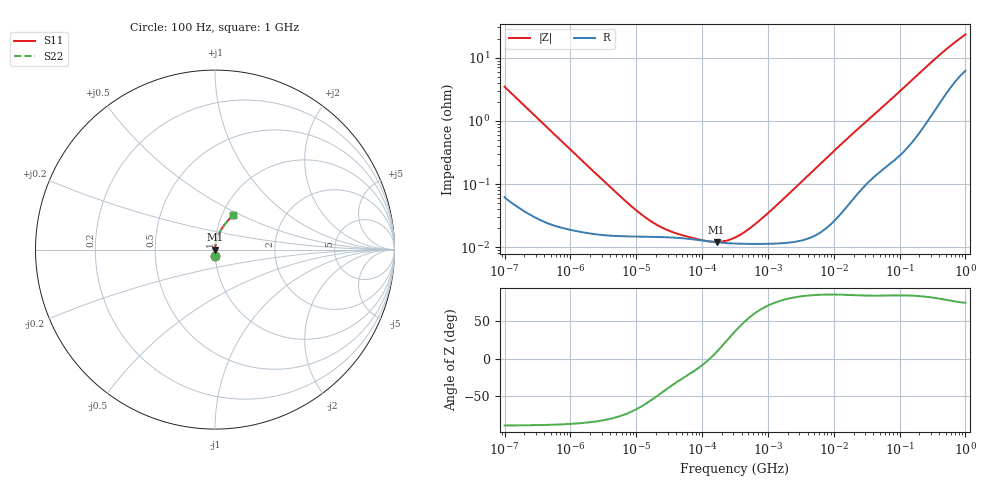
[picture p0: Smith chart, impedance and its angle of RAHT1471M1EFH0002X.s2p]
! RAHT1471M1EFH0002X  S-PARAMETER MODEL  (AEC-Q200 qualified)
! Model Generated by ELNA Corporation (http://www.ty-top.com)
! Version 1.0
! ELNA Control No. 201214
! Copyright (c) 2020 ELNA CO.,LTD. All Rights Reserved.
! Products Name : CONDUCTIVE POLYMER HYBRID ALUMINUM ELECTROLYTIC CAPACITORS
! Characteristics :
!  Capacitance  :  470uF  ,  Rated voltage  :  16V
!  Operating Temp. Range  :  -55 to +105 degC  ,  Endurance  :  5000hr at 105 degC
!  Dimension D  :  10mm  ,  Dimension L  :  10mm
! Frequency Range : 100Hz - 1GHz
! External Node Assignments :
!  1  o---| |---o  2
# MHz S RI R 50
!Freq[MHz].  S11 Real  S11 Imag  S21 Real  S21 Imag  S12 Real  S12 Imag  S22 Real  S22 Imag
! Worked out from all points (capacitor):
!   401 points, 100 Hz to 1 GHz, reference 50 ohm
!   read as one part in series: C = 461 uF near 108 Hz
!   lowest |Z| = 12.2 mohm at 166 kHz (marker M1)
!   series resonance near 131.1 kHz, so ESL is about 3.2 nH
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0.0001  0.00181 -0.0344  0.9982 0.0344  0.9982 0.0344  0.00181 -0.0344
0.000113  0.00149 -0.0305  0.9985 0.0305  0.9985 0.0305  0.00149 -0.0305
0.001488  0.000179 -0.00237  0.9998 0.00237  0.9998 0.00237  0.000179 -0.00237
0.00876  0.000148 -0.000406  0.9999 0.000406  0.9999 0.000406  0.000148 -0.000406
0.014207  0.000147 -0.00025  0.9999 0.00025  0.9999 0.00025  0.000147 -0.00025
0.022131  0.000146 -0.000161  0.9999 0.000161  0.9999 0.000161  0.000146 -0.000161
0.033113  0.000143 -0.000107  0.9999 0.000107  0.9999 0.000107  0.000143 -0.000107
0.055911  0.000138 -6.05e-05  0.9999 6.05e-05  0.9999 6.05e-05  0.000138 -6.05e-05
0.110917  0.000126 -1.24e-05  0.9999 1.24e-05  0.9999 1.24e-05  0.000126 -1.24e-05
0.165959  0.00012 1.9e-05  0.9999 -1.9e-05  0.9999 -1.9e-05  0.00012 1.9e-05
0.229087  0.000117 4.87e-05  0.9999 -4.87e-05  0.9999 -4.87e-05  0.000117 4.87e-05
0.316228  0.000115 8.49e-05  0.9999 -8.49e-05  0.9999 -8.49e-05  0.000115 8.49e-05
0.473151  0.000113 0.000144  0.9999 -0.000144  0.9999 -0.000144  0.000113 0.000144
0.767361  0.000113 0.000248  0.9999 -0.000248  0.9999 -0.000248  0.000113 0.000248
1.462177  0.000116 0.000484  0.9999 -0.000484  0.9999 -0.000484  0.000116 0.000484
4.704354  0.000148 0.00157  0.9999 -0.00157  0.9999 -0.00157  0.000148 0.00157
17.08048  0.000514 0.00553  0.9995 -0.00553  0.9995 -0.00553  0.000514 0.00553
69.9842  0.00246 0.0205  0.9975 -0.0205  0.9975 -0.0205  0.00246 0.0205
176.8072  0.00787 0.0494  0.9921 -0.0494  0.9921 -0.0494  0.00787 0.0494
395.8221  0.0286 0.1015  0.9714 -0.1015  0.9714 -0.1015  0.0286 0.1015
668.3439  0.0615 0.1492  0.9385 -0.1492  0.9385 -0.1492  0.0615 0.1492
1000  0.0984 0.1901  0.9016 -0.1901  0.9016 -0.1901  0.0984 0.1901
